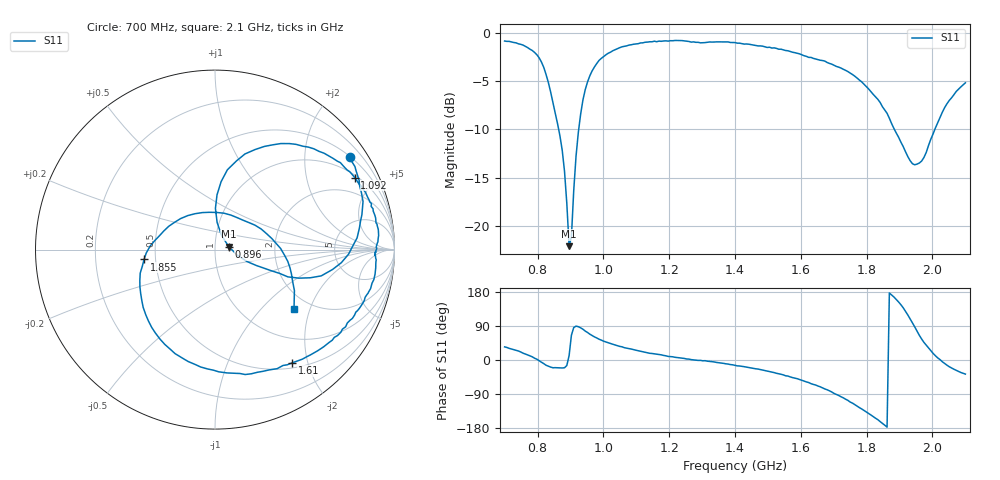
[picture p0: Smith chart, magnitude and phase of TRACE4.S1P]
! HP8714ET: E.06.01
! Reflection DATA:
# MHz  S  RI  R 50.0
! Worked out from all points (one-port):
!   201 points, 700 MHz to 2.1 GHz, reference 50 ohm
!   lowest |S11| = -22.1 dB at 896 MHz (marker M1), VSWR 1.17, Z = 58.3 + j1.88 ohm
!   |S11| at or under -10 dB: 864.3 MHz to 925.1 MHz (60.84 MHz wide, 6.8 % of centre); 1.884 GHz to 2.007 GHz (122.8 MHz wide, 6.31 % of centre)
!   S11 on the Smith chart (normalised r, x): 700 MHz: 0.52, +3.13; 896 MHz: 1.17, +0.04; 1.092 GHz: 1.11, +3.83; 1.61 GHz: 0.58, -1.75; 1.855 GHz: 0.43, -0.06; 2.1 GHz: 1.64, -1.57
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700  0.7494 0.5172
756  0.8247 0.2682
798  0.7719 0.0284
826  0.5919 -0.1464
875  0.2305 -0.0886
882  0.1798 -0.0671
896  0.0766 0.016
903  0.0363 0.0796
910  0.0118 0.1516
924  0.0113 0.3052
945  0.1204 0.4948
980  0.3675 0.5908
1050  0.6818 0.4926
1092  0.7793 0.4006
1225  0.9103 0.1043
1400  0.867 -0.2169
1505  0.7279 -0.4299
1575  0.5481 -0.5774
1610  0.4306 -0.6304
1673  0.1685 -0.696
1750  -0.2227 -0.5794
1806  -0.4003 -0.3212
1855  -0.3952 -0.0549
1925  -0.1106 0.2001
1967  0.1228 0.1784
2023  0.3657 0.00612
2051  0.4261 -0.1363
2100  0.4402 -0.3336
